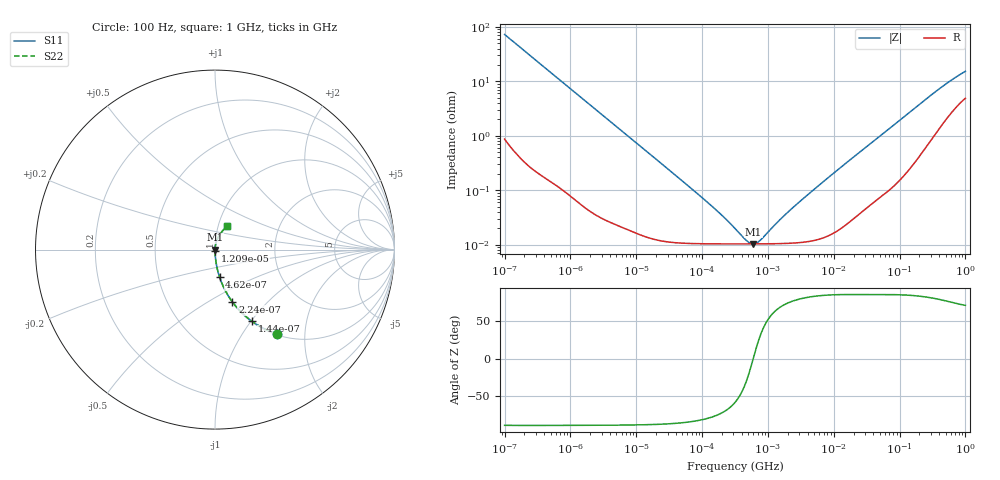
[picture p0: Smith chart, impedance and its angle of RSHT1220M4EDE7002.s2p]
! RSHT1220M4EDE7002  S-PARAMETER MODEL  (General Type)
! Model Generated by ELNA Corporation (http://www.ty-top.com)
! Version 1.0
! ELNA Control No.240229
! Copyright (c) 2024 ELNA CO.,LTD. All Rights Reserved.
! Products Name : CONDUCTIVE POLYMER HYBRID ALUMINUM ELECTROLYTIC CAPACITORS
! Characteristics :
!  Capacitance  :  22uF  ,  Rated voltage  :  63V
!  Operating Temp. Range  :  -55 to +105 degC  ,  Endurance  :  5000hr at 105 degC
!  Dimension D  :  6.3mm  ,  Dimension L  :  7.7mm
! Frequency Range : 100Hz - 1GHz
! External Node Assignments :
!  1  o---| |---o  2
# MHz S RI R 50
!Freq[MHz].  S11 Real  S11 Imag  S21 Real  S21 Imag  S12 Real  S12 Imag  S22 Real  S22 Imag
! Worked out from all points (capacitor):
!   401 points, 100 Hz to 1 GHz, reference 50 ohm
!   read as one part in series: C = 21.9 uF near 108 Hz
!   lowest |Z| = 10.4 mohm at 602.6 kHz (marker M1)
!   series resonance near 598.2 kHz, so ESL is about 3.2 nH
!   S11 on the Smith chart (normalised r, x): 100 Hz: 1.02, -1.45; 144 Hz: 1.01, -1.01; 224 Hz: 1.01, -0.65; 462 Hz: 1.00, -0.32; 12.09 kHz: 1.00, -0.01; 1 GHz: 1.10, +0.29
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0.0001  0.3471 -0.4701  0.6529 0.4701  0.6529 0.4701  0.3471 -0.4701
0.000144  0.2059 -0.3994  0.7941 0.3994  0.7941 0.3994  0.2059 -0.3994
0.000224  0.0975 -0.2922  0.9025 0.2922  0.9025 0.2922  0.0975 -0.2922
0.000462  0.0257 -0.1534  0.9743 0.1534  0.9743 0.1534  0.0257 -0.1534
0.000781  0.00966 -0.0927  0.9903 0.0927  0.9903 0.0927  0.00966 -0.0927
0.001488  0.00296 -0.0492  0.997 0.0492  0.997 0.0492  0.00296 -0.0492
0.012092  0.000186 -0.00614  0.9998 0.00614  0.9998 0.00614  0.000186 -0.00614
0.022131  0.000131 -0.00336  0.9999 0.00336  0.9999 0.00336  0.000131 -0.00336
0.130317  0.000104 -0.000545  0.9999 0.000545  0.9999 0.000545  0.000104 -0.000545
0.211349  0.000104 -0.000309  0.9999 0.000309  0.9999 0.000309  0.000104 -0.000309
0.316228  0.000103 -0.00017  0.9999 0.00017  0.9999 0.00017  0.000103 -0.00017
0.473151  0.000103 -5.9e-05  0.9999 5.9e-05  0.9999 5.9e-05  0.000103 -5.9e-05
0.533949  0.000104 -2.84e-05  0.9999 2.84e-05  0.9999 2.84e-05  0.000104 -2.84e-05
0.60256  0.000104 1.83e-06  0.9999 -1.83e-06  0.9999 -1.83e-06  0.000104 1.83e-06
0.679986  0.000104 3.21e-05  0.9999 -3.21e-05  0.9999 -3.21e-05  0.000104 3.21e-05
0.767361  0.000104 6.28e-05  0.9999 -6.28e-05  0.9999 -6.28e-05  0.000104 6.28e-05
1.788546  0.000106 0.000331  0.9999 -0.000331  0.9999 -0.000331  0.000106 0.000331
4.704354  0.000118 0.000964  0.9999 -0.000964  0.9999 -0.000964  0.000118 0.000964
69.9842  0.00119 0.0135  0.9988 -0.0135  0.9988 -0.0135  0.00119 0.0135
395.8221  0.0179 0.0687  0.9821 -0.0687  0.9821 -0.0687  0.0179 0.0687
668.3439  0.0399 0.1017  0.9601 -0.1017  0.9601 -0.1017  0.0399 0.1017
1000  0.0646 0.1294  0.9354 -0.1294  0.9354 -0.1294  0.0646 0.1294
